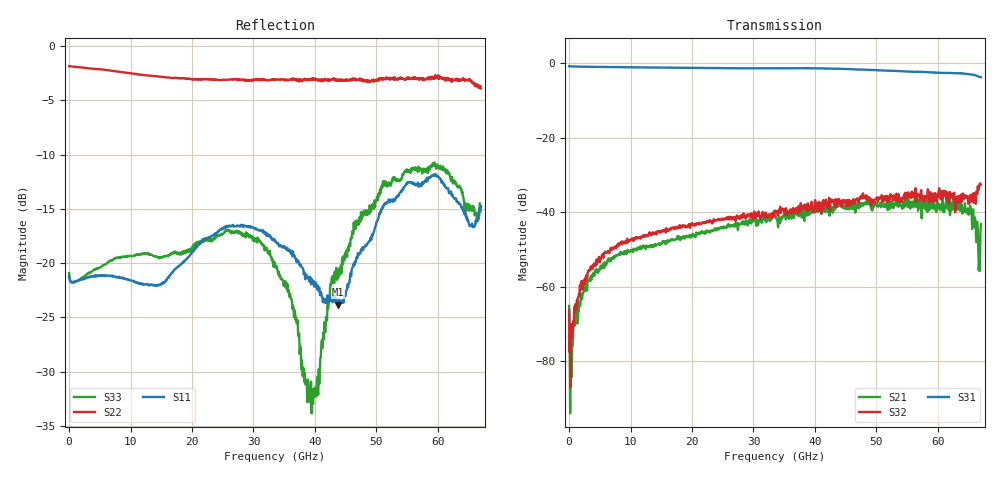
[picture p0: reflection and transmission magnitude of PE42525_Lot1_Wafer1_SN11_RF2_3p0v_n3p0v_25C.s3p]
!Keysight Technologies,N5227A,US51270237,A.10.43.00
!Date: Friday, September 16, 2016 08:59:17
!Correction: S11(Full 3 Port(1,2,3))
!S12(Full 3 Port(1,2,3))
!S13(Full 3 Port(1,2,3))
!S21(Full 3 Port(1,2,3))
!S22(Full 3 Port(1,2,3))
!S23(Full 3 Port(1,2,3))
!S31(Full 3 Port(1,2,3))
!S32(Full 3 Port(1,2,3))
!S33(Full 3 Port(1,2,3))
!S3P File: Measurements: <S11,S12,S13>,
!<S21,S22,S23>,
!<S31,S32,S33>:
# Hz S  dB  R 50
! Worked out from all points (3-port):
!   801 points, 10 MHz to 67 GHz, reference 50 ohm
!   strongest paths, dB at 10 MHz, 16.76 GHz, 33.51 GHz, 50.25 GHz, 67 GHz:
!     S31: -0.9, -1.3, -1.4, -2.0, -3.8
!     S32: -66.3, -44.2, -39.9, -37.2, -32.6
!     S21: -65.2, -47.6, -41.1, -38.1, -43.3
!   lowest |S11| = -23.8 dB at 43.8 GHz (marker M1), VSWR 1.14, Z = 44.8 - j3.19 ohm
!   |S11| at or under -10 dB: start of sweep to end of sweep
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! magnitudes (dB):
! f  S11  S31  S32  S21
! 10 MHz  -21.1  -0.9  -66.3  -65.2
! 428.7 MHz  -21.7  -0.9  -73.8  -84.3
! 3.025 GHz  -21.3  -1.0  -56.6  -58.4
! 8.216 GHz  -21.3  -1.1  -48.5  -51.4
! 33.51 GHz  -18.0  -1.4  -39.9  -41.1
! 39.62 GHz  -21.9  -1.4  -39.6  -38.5
! 43.8 GHz  -23.8  -1.5  -37.7  -37.5
! 55.11 GHz  -12.6  -2.3  -36.3  -38.6
! 64.57 GHz  -15.8  -2.9  -36.1  -39.8
! 67 GHz  -14.8  -3.8  -32.6  -43.3
